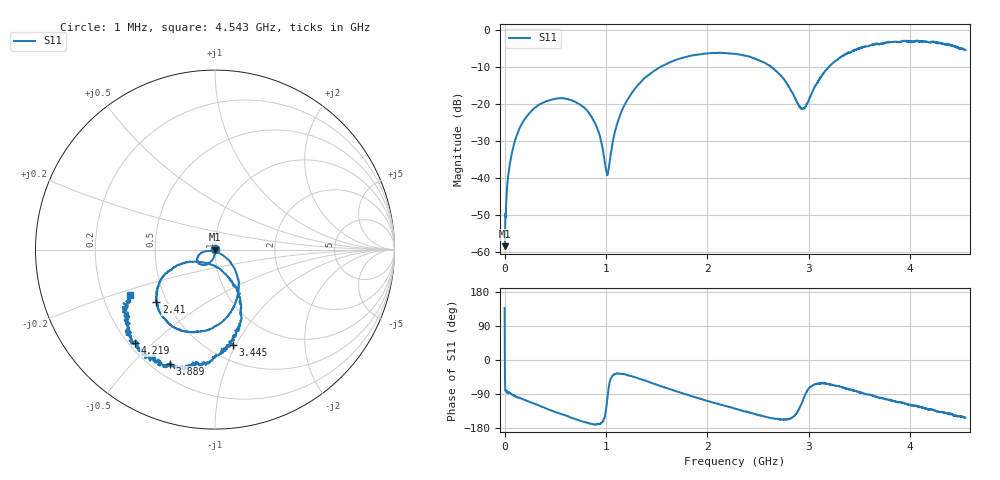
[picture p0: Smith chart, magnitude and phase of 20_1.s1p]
# HZ S RI R 50
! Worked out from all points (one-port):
!   1515 points, 1 MHz to 4.543 GHz, reference 50 ohm
!   lowest |S11| = -58.4 dB at 4 MHz (marker M1), VSWR 1.00, Z = 50.1 - j0.0759 ohm
!   |S11| at or under -10 dB: start of sweep to 1.538 GHz; 2.631 GHz to 3.196 GHz (565.1 MHz wide, 19.4 % of centre)
!   S11 on the Smith chart (normalised r, x): 1 MHz: 1.00, +0.00; 2.41 GHz: 0.44, -0.32; 3.445 GHz: 0.65, -0.97; 3.889 GHz: 0.27, -0.64; 4.219 GHz: 0.22, -0.44; 4.543 GHz: 0.32, -0.22
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1000000  -0.000953 0.000883
4000000  0.000932 -0.000758
3.1e7  0.00103 -0.00885
5.2e7  0.00105 -0.0152
9.1e7  -0.00125 -0.0279
1.48e8  -0.0078 -0.0463
3.19e8  -0.0432 -0.0825
5.71e8  -0.0966 -0.0709
8.53e8  -0.067 -0.014
9.31e8  -0.0401 -0.00765
1.012e9  -0.00296 -0.0105
1.087e9  0.0329 -0.0247
1.138e9  0.0563 -0.0405
1.372e9  0.1311 -0.1747
1.705e9  0.0461 -0.3972
1.978e9  -0.1352 -0.4586
2.272e9  -0.2934 -0.3715
2.41e9  -0.3262 -0.2913
2.641e9  -0.2755 -0.1353
2.842e9  -0.1197 -0.0678
2.953e9  -0.0143 -0.0878
3.172e9  0.1281 -0.2573
3.409e9  0.1067 -0.4799
3.445e9  0.0983 -0.5301
3.889e9  -0.2525 -0.6346
3.976e9  -0.3165 -0.6182
4.219e9  -0.4477 -0.5217
4.543e9  -0.4724 -0.2507
